(* Logix 5000 AddOnInstructionDefinition export TSx_AOI_8P; software revision 33.00 *)

ADD_ON_INSTRUCTION TSx_AOI_8P   (* revision 1.0, vendor PM Controls *)
// Anderson-Negele Temperature Sensor
// Revision note:
// psm
VAR_OUTPUT
   IOLink_Mode : BOOL; {access Read Only, visible}
   Device_Not_Connected : BOOL; {access Read Only, visible}
END_VAR
VAR_IN_OUT
   Input : INT[223]; {required}
END_VAR
VAR_INPUT
   Port_Process_Data_Size : INT := 4;
   Port_Number : INT; {visible}
   Temp_Value_Gradient : REAL := 0.01;
END_VAR
VAR_OUTPUT
   Vendor_ID : INT; {access Read Only, visible}
   Device_ID : INT; {access Read Only, visible}
   Invalid_Data : BOOL; {access Read Only, visible}
   Temperature : REAL; {access Read Only, visible}
END_VAR
VAR
   StatusFlgs_Offset : INT; {access None}
   RealPort_Num : INT; {access None}
   Process_PDI : INT; {access None}
   Process_Offset : INT; {access None}
   Offset_StatusFlgs : INT; {access None}
   Offset_Address : INT; {access None}
   Data_Size : INT; {access None}
   Temp_DINT : DINT; {access None}
END_VAR

ROUTINE Logic   (* ladder *)
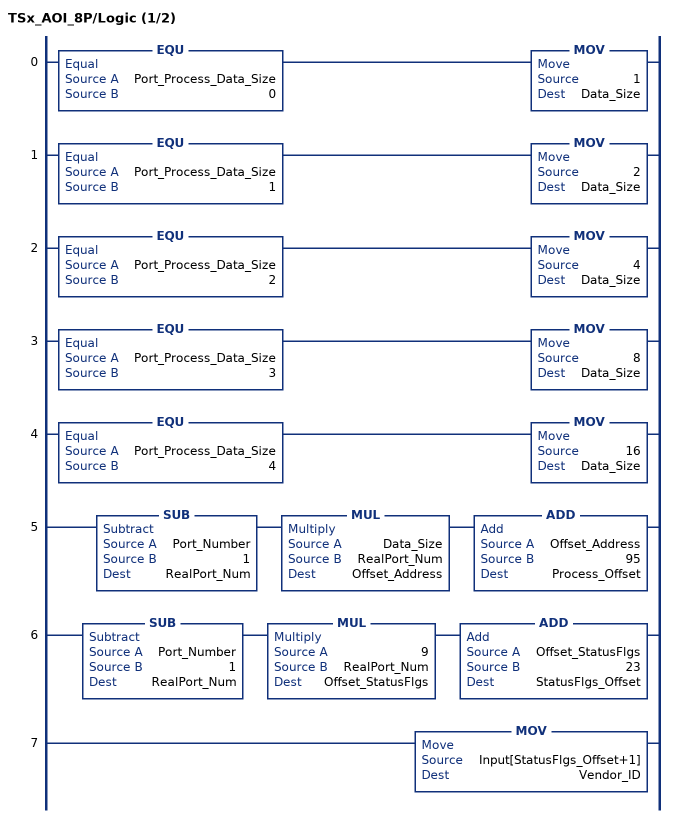
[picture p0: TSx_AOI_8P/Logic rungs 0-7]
   0: EQU(Port_Process_Data_Size,0)MOV(1,Data_Size);
   1: EQU(Port_Process_Data_Size,1)MOV(2,Data_Size);
   2: EQU(Port_Process_Data_Size,2)MOV(4,Data_Size);
   3: EQU(Port_Process_Data_Size,3)MOV(8,Data_Size);
   4: EQU(Port_Process_Data_Size,4)MOV(16,Data_Size);
   5: SUB(Port_Number,1,RealPort_Num)MUL(Data_Size,RealPort_Num,Offset_Address)ADD(Offset_Address,95,Process_Offset);
   6: SUB(Port_Number,1,RealPort_Num)MUL(9,RealPort_Num,Offset_StatusFlgs)ADD(Offset_StatusFlgs,23,StatusFlgs_Offset);
   7: MOV(Input[StatusFlgs_Offset+1],Vendor_ID);
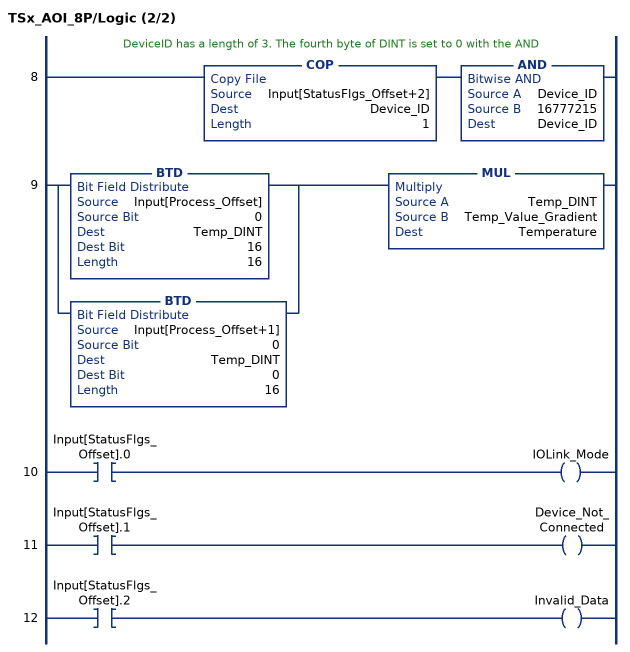
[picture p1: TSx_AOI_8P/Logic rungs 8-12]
   // DeviceID has a length of 3. The fourth byte of DINT is set to 0 with the AND
   8: COP(Input[StatusFlgs_Offset+2],Device_ID,1)AND(Device_ID,16777215,Device_ID);
   9: [BTD(Input[Process_Offset],0,Temp_DINT,16,16) ,BTD(Input[Process_Offset+1],0,Temp_DINT,0,16) ]MUL(Temp_DINT,Temp_Value_Gradient,Temperature);
   10: XIC(Input[StatusFlgs_Offset].0)OTE(IOLink_Mode);
   11: XIC(Input[StatusFlgs_Offset].1)OTE(Device_Not_Connected);
   12: XIC(Input[StatusFlgs_Offset].2)OTE(Invalid_Data);
END_ROUTINE
END_ADD_ON_INSTRUCTION
